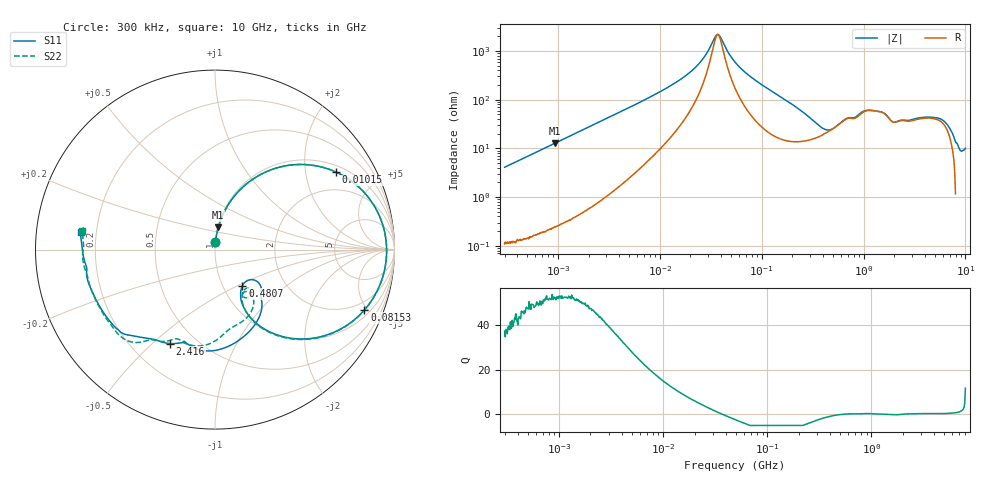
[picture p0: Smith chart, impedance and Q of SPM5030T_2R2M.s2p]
! S-Parameter Data Generated by TDK Corporation
! Copyright(C) 2019 TDK Corporation.
! All Rights Reserved.
! TDK P/N: SPM5030T-2R2M (Inductor)
! Property: L=2.2uH at 100kHz
! Size(LxWxT): 5.2x5x3mm
! Model Type: s2p (Touchstone File Format Version 1.0)
! Frequency: DC=Yes Start=0.3MHz Stop=10000MHz 802points Log-sweep
! Model Generated on Sep. 23, 2019
! Port Assignments:
!  1 ---@@@--- 2
! Applicable Conditions:
!  Temperature = 25 degC
!  DC Bias Current = 0 A
!  Small Signal Operation
! Terms and conditions regarding TDK Simulation Models
! (1)This simulation model is being provided solely for informational purposes. Please refer to the specifications of the products in terms of detailed characteristics of such products.
! (2)In no event shall TDK Corporation of any of its subsidiaries be liable for any loss or damage arising, directly or indirectly,
!  From any information contained in this simulation model, including, but not limited to loss or damages arising from any inaccuracies, omissions or errors in connection with such information.
! (3)Any and all copyrights on this simulation model are owned by TDK Corporation.
!  Duplication or redistribution of this simulation model without prior written permission from TDK Corporation is prohibited.
! (4)This simulation model is subject to any modification or change without any prior notice.
! (5)Neither TDK Corporation nor any of its subsidiaries shall make any warranty, express or implied,
!  Including but not limited to the correctness, implied warranties of merchantability and fitness for a particular purpose with respect to this simulation models.
! (6)The use of this simulation model shall be deemed to have consented to the terms and conditions hereof.
# Hz S MA R 50
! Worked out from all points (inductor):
!   801 points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, 300 kHz to 10 GHz, reference 50 ohm
!   read as one part in series: L = 2.17 uH near 318.3 kHz
!   highest Q = 52.8 at 930.3 kHz (marker M1), where L = 2.17 uH
!   self-resonance near 37.14 MHz
!   S11 on the Smith chart (normalised r, x): 300 kHz: 1.00, +0.08; 10.15 MHz: 1.23, +2.96; 81.53 MHz: 1.37, -4.76; 480.7 MHz: 1.23, -0.53; 2.416 GHz: 0.36, -0.57; 10 GHz: 0.14, +0.07
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300000  0.04052 86.1  0.998 -2.4  0.9982 -2.4  0.04055 86.1
930288  0.1251 81.6  0.9898 -7.2  0.9896 -7.2  0.1251 81.7
1713600  0.2256 75.7  0.9696 -13.1  0.9698 -13.1  0.2256 75.7
3822232  0.4567 61.0  0.8763 -27.3  0.8763 -27.3  0.4567 61.0
9671944  0.788 34.0  0.5669 -52.3  0.567 -52.3  0.788 34.0
1.014698e7  0.8016 32.6  0.546 -53.6  0.546 -53.6  0.8017 32.6
2.220835e7  0.9378 10.7  0.207 -67.7  0.207 -67.7  0.9379 10.7
3.686242e7  0.9563 -1.4  0.04376 -5.2  0.04376 -5.3  0.9564 -1.5
5.477226e7  0.9423 -11.1  0.1582 62.0  0.1583 62.0  0.9425 -11.2
8.153051e7  0.8977 -22.0  0.3219 58.9  0.3219 58.9  0.8981 -22.2
1.630679e8  0.701 -45.3  0.6247 37.0  0.6248 37.0  0.7024 -45.5
3.126428e8  0.4015 -63.1  0.7973 9.0  0.7974 9.0  0.4093 -63.1
4.807079e8  0.2526 -52.8  0.7844 -10.2  0.7845 -10.2  0.2786 -55.0
6.573376e8  0.2911 -37.1  0.6972 -22.1  0.6972 -22.1  0.3152 -50.2
8.414386e8  0.3614 -45.2  0.666 -28.8  0.666 -28.8  0.2876 -54.6
1.054047e9  0.4417 -55.3  0.5778 -35.9  0.5778 -35.9  0.3974 -59.1
1.767019e9  0.5616 -101.3  0.525 -44.0  0.5251 -44.0  0.5382 -96.8
2.416286e9  0.5798 -115.5  0.4853 -65.9  0.4855 -65.9  0.5698 -117.0
4.34106e9  0.6867 -136.5  0.2985 -95.4  0.2986 -95.5  0.7044 -133.9
6.010849e9  0.7067 -143.7  0.2432 -111.6  0.2433 -111.6  0.7173 -148.5
8.770142e9  0.7346 -177.0  0.1718 -144.6  0.1717 -144.7  0.7407 174.1
1e10  0.7546 172.4  0.1408 -152.5  0.1408 -152.6  0.746 172.2
